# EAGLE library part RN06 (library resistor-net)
RESISTOR NETWORK
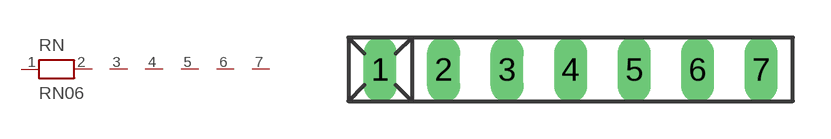
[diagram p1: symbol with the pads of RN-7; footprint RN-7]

Designator prefix RN

## RN06 (OC_FARNELL: unknown; OC_NEWARK: unknown)  [RN-7]
1  1  pas
2  2  pas
3  3  pas
4  4  pas
5  5  pas
6  6  pas
7  7  pas

## Footprint RN-7 (pad centres in mm)
RESISTOR NETWORK
drill 0.813 long: 1 -7.62,0; 2 -5.08,0; 3 -2.54,0; 4 0,0; 5 2.54,0; 6 5.08,0; 7 7.62,0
